|Texas Instruments Incorporated
|tmux5412, 4 Data Lane 1:1 50V Switch
[IBIS Ver]   4.1
[File name]   tmux5412.ibs
[Date]   04/29/25
[File Rev]   1.0
[Source]
| Texas Instruments Incorporated.
| ASC-INT-MPD
| 12500 TI Blvd
| Dallas, TX - 75243
[Notes]   Revision History:
| Rev 1.0: 04/29/25
| - Initial version of the model
| - Model generated from simulations in SPECTRE
| - C_comp although listed in numerical order of value are
|   obtained from varying PVT conditions. For PVT conditions for
|   each specific value refer the buffer description under
|   respective [Model]. IBIS model user is responsible for using
|   appropriate C_comp to simulate for Signal Integrity.
[Disclaimer]
| This model is designed as an aid for customers of Texas Instruments.
| TI and its licensors and suppliers make no warranties, either expressed
| or implied, with respect to this  model, including the warranties of
| merchantability or fitness for a particular purpose. The model is
| provided solely on an "as is" basis. The entire risk as to its quality
| and performance is with the customer.
| This model is subject to change without notice. Texas Instruments
| Incorporated is not responsible for updating this model.
[Copyright]
(C) Copyright 2025 Texas Instruments Incorporated.All rights reserved.
|  Component TMUX5412PW 16-pin - PW package
|  Part # TMUX5412PW
[Component]   TMUX5412PW
[Manufacturer]  TI
[Package]
|   typ   min   max
R_pkg   0.0668   NA   NA
L_pkg   2.1992nH   NA   NA
C_pkg   0.2884pF   NA   NA
[Pin]   signal_name   model_name
   1   SEL1   inbuf
   2   D1   dterm
   3   S1   sterm
   4   VSS   power
   5   GND   gnd
   6   S4   sterm
   7   D4   dterm
   8   SEL4   inbuf
   9   SEL3   inbuf
   10   D3   dterm
   11   S3   sterm
   12   NC   nc
   13   VDD   power
   14   S2   sterm
   15   D2   dterm
   16   SEL2   inbuf
[Series Switch Groups]
On 1 /
On 2 /
On 3 /
On 4 /
Off 1 /
[Series Pin Mapping]  pin_2 model_name function_table_group
   3   2   switch_dual_15   1
  14  15   switch_dual_15   1
  11  10   switch_dual_15   1
   6   7   switch_dual_15   1
|   3   2   switch_36   1
|  14  15   switch_36   1
|  11  10   switch_36   1
|   6   7   switch_36   1
|   3   2   switch_12   1
|  14  15   switch_12   1
|  11  10   switch_12   1
|   6   7   switch_12   1
|   3   2   switch_48   1
|  14  15   switch_48   1
|  11  10   switch_48   1
|   6   7   switch_48   1
|   3   2   switch_dual_20   1
|  14  15   switch_dual_20   1
|  11  10   switch_dual_20   1
|   6   7   switch_dual_20   1
|   3   2   switch_dual_25   1
|  14  15   switch_dual_25   1
|  11  10   switch_dual_25   1
|   6   7   switch_dual_25   1
|   3   2   switch_5   1
|  14  15   switch_5   1
|  11  10   switch_5   1
|   6   7   switch_5   1
|  Component TMUX5412DYY 16-pin - DYY package
|  Part # TMUX5412DYY
[Component]   TMUX5412DYY
[Manufacturer]  TI
[Package]
|   typ   min   max
R_pkg   0.0668   NA   NA
L_pkg   2.1992nH   NA   NA
C_pkg   0.2884pF   NA   NA
[Pin]   signal_name   model_name
   1   SEL1   inbuf
   2   D1   dterm
   3   S1   sterm
   4   VSS   power
   5   GND   gnd
   6   S4   sterm
   7   D4   dterm
   8   SEL4   inbuf
   9   SEL3   inbuf
   10   D3   dterm
   11   S3   sterm
   12   NC   nc
   13   VDD   power
   14   S2   sterm
   15   D2   dterm
   16   SEL2   inbuf
[Series Switch Groups]
On 1 /
On 2 /
On 3 /
On 4 /
Off 1 /
[Series Pin Mapping]  pin_2 model_name function_table_group
   3   2   switch_dual_15   1
  14  15   switch_dual_15   1
  11  10   switch_dual_15   1
   6   7   switch_dual_15   1
|   3   2   switch_36   1
|  14  15   switch_36   1
|  11  10   switch_36   1
|   6   7   switch_36   1
|   3   2   switch_12   1
|  14  15   switch_12   1
|  11  10   switch_12   1
|   6   7   switch_12   1
|   3   2   switch_48   1
|  14  15   switch_48   1
|  11  10   switch_48   1
|   6   7   switch_48   1
|   3   2   switch_dual_20   1
|  14  15   switch_dual_20   1
|  11  10   switch_dual_20   1
|   6   7   switch_dual_20   1
|   3   2   switch_dual_25   1
|  14  15   switch_dual_25   1
|  11  10   switch_dual_25   1
|   6   7   switch_dual_25   1
|   3   2   switch_5   1
|  14  15   switch_5   1
|  11  10   switch_5   1
|   6   7   switch_5   1
[Model Selector] dterm
dterm_dual_15 Use for operation at +/-15V
dterm_36 Use for operation at 36V
dterm_12 Use for operation at 12V
dterm_48 Use for operation at 48V
dterm_dual_20 Use for operation at +/-20V
dterm_dual_25 Use for operation at +/-25V
dterm_5 Use for operation at 5V
[Model Selector] sterm
sterm_dual_15 Use for operation at +/-15V
sterm_36 Use for operation at 36V
sterm_12 Use for operation at 12V
sterm_48 Use for operation at 48V
sterm_dual_20 Use for operation at +/-20V
sterm_dual_25 Use for operation at +/-25V
sterm_5 Use for operation at 5V
[Model Selector] inbuf
inbuf_dual_15 Use for operation at +/-15V
inbuf_36 Use for operation at 36V
inbuf_12 Use for operation at 12V
inbuf_48 Use for operation at 48V
inbuf_dual_20 Use for operation at +/-20V
inbuf_dual_25 Use for operation at +/-25V
inbuf_5 Use for operation at 5V
| switch_dual_15
[Model]   switch_dual_15
Model_type   Series_switch
|   typ   min   max
C_comp   1.008417e-11   NA   NA
[Voltage Range]   15   NA   NA
[Power Clamp Reference]   15   NA   NA
[Temperature Range]   27   NA   NA
[On]
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[Off]
|   typ   min   max
[R Series]   10G   NA   NA
| switch_36
[Model]   switch_36
Model_type   Series_switch
|   typ   min   max
C_comp   1.008417e-11   NA   NA
[Voltage Range]   36   NA   NA
[Power Clamp Reference]   36   NA   NA
[Temperature Range]   27   NA   NA
[On]
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[Off]
|   typ   min   max
[R Series]   10G   NA   NA
| switch_12
[Model]   switch_12
Model_type   Series_switch
|   typ   min   max
C_comp   1.008417e-11   NA   NA
[Voltage Range]   12   NA   NA
[Power Clamp Reference]   12   NA   NA
[Temperature Range]   27   NA   NA
[On]
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[Off]
|   typ   min   max
[R Series]   10G   NA   NA
| switch_48
[Model]   switch_48
Model_type   Series_switch
|   typ   min   max
C_comp   1.008417e-11   NA   NA
[Voltage Range]   48   NA   NA
[Power Clamp Reference]   48   NA   NA
[Temperature Range]   27   NA   NA
[On]
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[Off]
|   typ   min   max
[R Series]   10G   NA   NA
| switch_dual_20
[Model]   switch_dual_20
Model_type   Series_switch
|   typ   min   max
C_comp   1.008417e-11   NA   NA
[Voltage Range]   20   NA   NA
[Power Clamp Reference]   20   NA   NA
[Temperature Range]   27   NA   NA
[On]
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[Off]
|   typ   min   max
[R Series]   10G   NA   NA
| switch_dual_25
[Model]   switch_dual_25
Model_type   Series_switch
|   typ   min   max
C_comp   1.008417e-11   NA   NA
[Voltage Range]   25   NA   NA
[Power Clamp Reference]   25   NA   NA
[Temperature Range]   27   NA   NA
[On]
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[Off]
|   typ   min   max
[R Series]   10G   NA   NA
| switch_5
[Model]   switch_5
Model_type   Series_switch
|   typ   min   max
C_comp   1.008417e-11   NA   NA
[Voltage Range]   5   NA   NA
[Power Clamp Reference]   5   NA   NA
[Temperature Range]   27   NA   NA
[On]
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[Off]
|   typ   min   max
[R Series]   10G   NA   NA
| Models and submodels in the file (28): dterm_dual_15 (Terminator), dterm_36 (Terminator), dterm_12 (Terminator), dterm_48 (Terminator), dterm_dual_20 (Terminator), dterm_dual_25 (Terminator), dterm_5 (Terminator), switch_dual_15 (Series_switch), switch_36 (Series_switch), switch_12 (Series_switch), switch_48 (Series_switch), switch_dual_20 (Series_switch), switch_dual_25 (Series_switch), switch_5 (Series_switch), sterm_dual_15 (Terminator), sterm_36 (Terminator), sterm_12 (Terminator), sterm_48 (Terminator), sterm_dual_20 (Terminator), sterm_dual_25 (Terminator), sterm_5 (Terminator), inbuf_dual_15 (Input), inbuf_36 (Input), inbuf_12 (Input), inbuf_48 (Input), inbuf_dual_20 (Input), inbuf_dual_25 (Input), inbuf_5 (Input)
